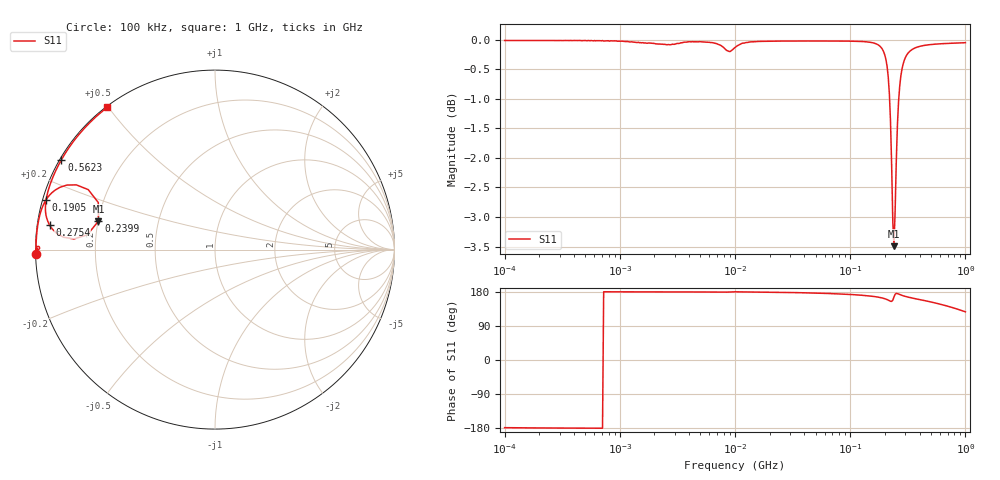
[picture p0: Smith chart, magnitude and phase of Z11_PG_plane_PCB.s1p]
!1 port Z parameter measurement of a P-G plane of a PCB
# HZ Z MA R 50
!freq magS11 phS11
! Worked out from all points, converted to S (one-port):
!   401 points, 100 kHz to 1 GHz, reference 50 ohm
!   lowest |S11| = -3.5 dB at 239.9 MHz (marker M1), VSWR 5.04, Z = 10.1 + j5.77 ohm
!   |S11| at or under -10 dB: nowhere
!   S11 on the Smith chart (normalised r, x): 100 kHz: 0.00, -0.01; 190.5 MHz: 0.01, +0.14; 239.9 MHz: 0.20, +0.12; 275.4 MHz: 0.04, +0.07; 562.3 MHz: 0.00, +0.27; 1 GHz: 0.00, +0.50
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100000  0.0128 -86.1
316227.8  0.003901 -75.9
1000000  0.001924 42.3
3162278  0.003723 9.0
7762471  0.01139 53.4
1e7  0.007714 3.0
3.162278e7  0.01838 85.6
5.888437e7  0.0356 87.8
1.023293e8  0.06336 88.6
1.513561e8  0.1002 88.4
1.905461e8  0.1445 86.2
2.041738e8  0.1707 83.3
2.137962e8  0.197 79.0
2.187762e8  0.215 75.2
2.238721e8  0.2358 69.2
2.290868e8  0.2559 59.8
2.344229e8  0.2617 45.9
2.398833e8  0.232 29.8
2.511886e8  0.1244 17.4
2.570396e8  0.09233 26.0
2.630268e8  0.07887 40.4
2.754229e8  0.08157 64.3
2.884032e8  0.09576 75.6
3.162278e8  0.1224 83.6
4.168694e8  0.1909 88.1
5.623413e8  0.2713 89.0
7.413102e8  0.3648 89.4
1e9  0.4974 89.6
